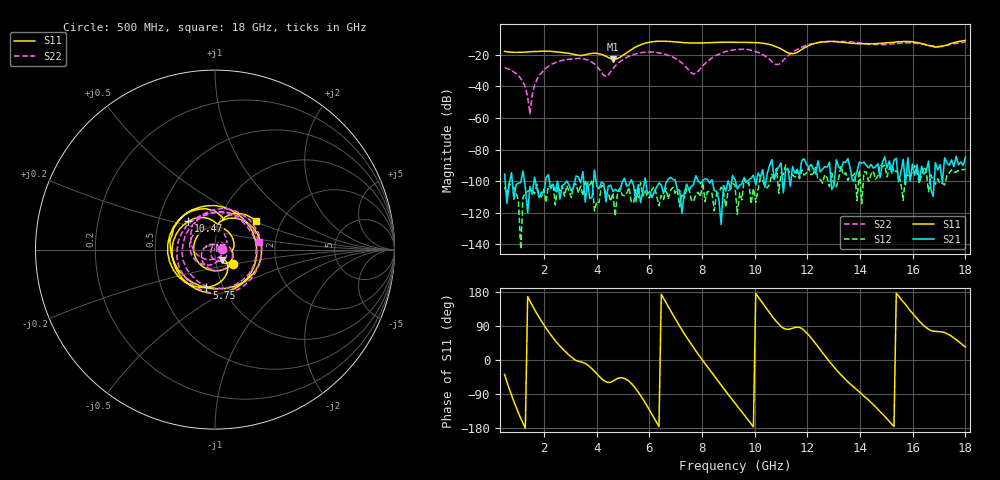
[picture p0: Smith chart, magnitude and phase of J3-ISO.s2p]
!Agilent Technologies,N5230A,MY45001360,A.07.50.67
!Agilent N5230A: A.07.50.67
!Date: Tuesday, April 16, 2024 15:53:06
!Correction: S11(Full 2 Port(1,2))
!S21(Full 2 Port(1,2))
!S12(Full 2 Port(1,2))
!S22(Full 2 Port(1,2))
!S2P File: Measurements: S11, S21, S12, S22:
# Hz S  dB  R 50
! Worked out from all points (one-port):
!   201 points, 500 MHz to 18 GHz, reference 50 ohm
!   lowest |S11| = -23.0 dB at 4.612 GHz (marker M1), VSWR 1.15, Z = 53.8 - j6.33 ohm
!   |S11| at or under -10 dB: start of sweep to end of sweep
!   S11 on the Smith chart (normalised r, x): 500 MHz: 1.20, -0.19; 5.75 GHz: 0.83, -0.37; 10.47 GHz: 0.71, +0.24; 18 GHz: 1.50, +0.51
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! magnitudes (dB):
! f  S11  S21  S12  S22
! 500 MHz  -18.0  -95.6  -103.8  -28.4
! 1.2 GHz  -18.6  -93.7  -110.3  -37.6
! 1.288 GHz  -18.5  -104.0  -107.4  -40.4
! 1.462 GHz  -18.3  -103.4  -105.6  -57.5
! 1.55 GHz  -18.2  -108.2  -105.6  -45.5
! 1.637 GHz  -18.1  -97.5  -108.1  -39.3
! 1.988 GHz  -17.9  -107.5  -105.3  -30.0
! 3.475 GHz  -20.4  -94.0  -109.3  -22.6
! 4.35 GHz  -21.1  -113.1  -107.7  -33.9
! 4.612 GHz  -23.0  -106.6  -107.5  -28.9
! 5.75 GHz  -13.3  -106.6  -109.4  -18.7
! 6.362 GHz  -11.6  -101.1  -115.6  -18.9
! 7.675 GHz  -12.7  -102.1  -112.9  -32.3
! 8.463 GHz  -12.4  -106.1  -118.7  -21.2
! 9.25 GHz  -12.2  -99.1  -102.3  -16.9
! 10.47 GHz  -13.3  -95.1  -104.3  -21.9
! 10.91 GHz  -15.7  -91.0  -107.6  -26.1
! 11.44 GHz  -19.5  -90.7  -96.1  -18.4
! 12.22 GHz  -13.2  -92.4  -95.2  -13.0
! 15.11 GHz  -12.5  -87.2  -92.0  -13.4
! 16.86 GHz  -15.4  -88.3  -101.8  -14.6
! 18 GHz  -11.1  -84.8  -92.4  -12.1
